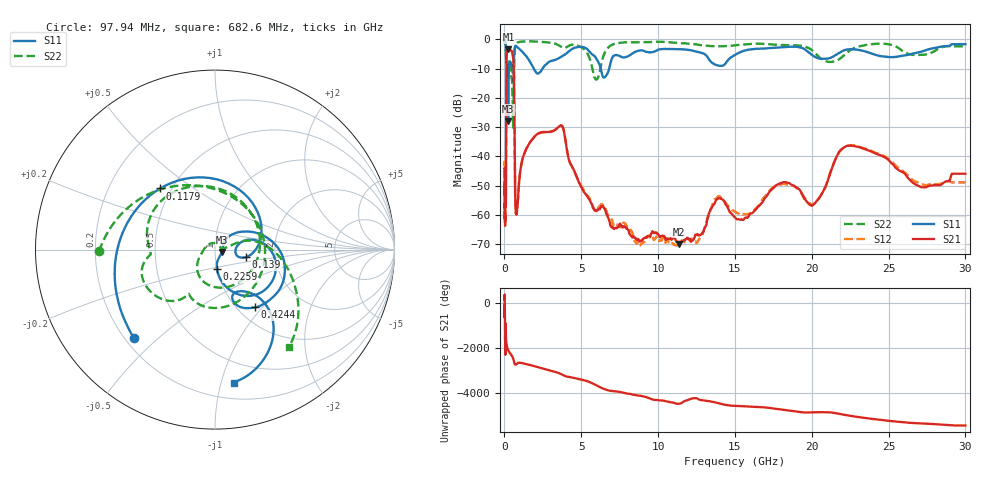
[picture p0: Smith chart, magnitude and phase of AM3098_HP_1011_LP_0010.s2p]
! Date/Time: Thu, Feb 28, 2019 8:42 AM
! Network Analyzer: Agilent Technologies E8364B Rev: A.07.50.67
! Sweep from 0.010 to 30.000 GHz, 1601 Points, Sweep Type: LOG
! Power Supply: 5.022 V, 0.002 A
# Hz S DB R 50
!freq MagS11 AngS11 MagS21 AngS21 MagS12 AngS12 MagS22 AngS22
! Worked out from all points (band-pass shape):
!   1601 points, 10 MHz to 30 GHz, reference 50 ohm
!   highest |S21| = -3.40 dB at 261.2 MHz (marker M1); lowest = -70.0 dB at 11.36 GHz (marker M2)
!   |S21| within 3 dB of the highest: 136.7 MHz to 567.5 MHz (430.8 MHz wide, 122 % of centre)
!   lowest |S11| = -28.0 dB at 239.9 MHz (marker M3), VSWR 1.08, Z = 53.9 - j1.47 ohm
!   |S11| at or under -10 dB: 200.2 MHz to 293.5 MHz (93.28 MHz wide, 37.8 % of centre); 1.909 GHz to 2.475 GHz (566 MHz wide, 25.8 % of centre); 6.27 GHz to 6.817 GHz (546.3 MHz wide, 8.35 % of centre)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
!   |S22| runs from -30.2 to -0.5 dB; largest |S21 - S12| = 0.012
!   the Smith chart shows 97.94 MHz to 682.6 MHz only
!   S11 on the Smith chart (normalised r, x): 97.94 MHz: 0.24, -0.42; 117.9 MHz: 0.43, +0.37; 139 MHz: 1.41, -0.12; 225.9 MHz: 1.00, -0.22; 424.4 MHz: 1.20, -0.91; 682.6 MHz: 0.33, -1.10
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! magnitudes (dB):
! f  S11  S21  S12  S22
! 10 MHz  -0.3  -43.9  -43.4  -0.5
! 38.04 MHz  -0.4  -61.0  -60.8  -0.7
! 97.94 MHz  -3.5  -52.6  -52.2  -3.8
! 117.9 MHz  -6.8  -20.6  -20.6  -10.7
! 139 MHz  -15.0  -5.9  -5.8  -10.6
! 144.7 MHz  -18.3  -5.1  -5.1  -10.8
! 225.9 MHz  -19.2  -3.5  -3.4  -8.7
! 239.9 MHz  -28.0  -3.4  -3.4  -8.9
! 261.2 MHz  -16.3  -3.4  -3.3  -8.7
! 424.4 MHz  -8.2  -3.7  -3.7  -11.8
! 550.5 MHz  -11.5  -5.6  -5.5  -28.6
! 617.6 MHz  -6.2  -13.5  -13.4  -13.7
! 682.6 MHz  -2.5  -46.3  -46.5  -3.3
! 785.3 MHz  -2.4  -59.6  -57.2  -1.4
! 2.084 GHz  -11.5  -32.6  -32.6  -0.7
! 3.723 GHz  -5.8  -29.5  -29.5  -2.6
! 5.989 GHz  -6.6  -58.7  -58.8  -13.7
! 7.926 GHz  -6.0  -64.7  -64.1  -1.0
! 11.36 GHz  -3.3  -70.0  -69.2  -1.2
! 20.2 GHz  -5.9  -56.1  -55.9  -4.6
! 22.67 GHz  -3.4  -36.4  -36.2  -3.2
! 30 GHz  -1.6  -45.9  -48.9  -2.3
